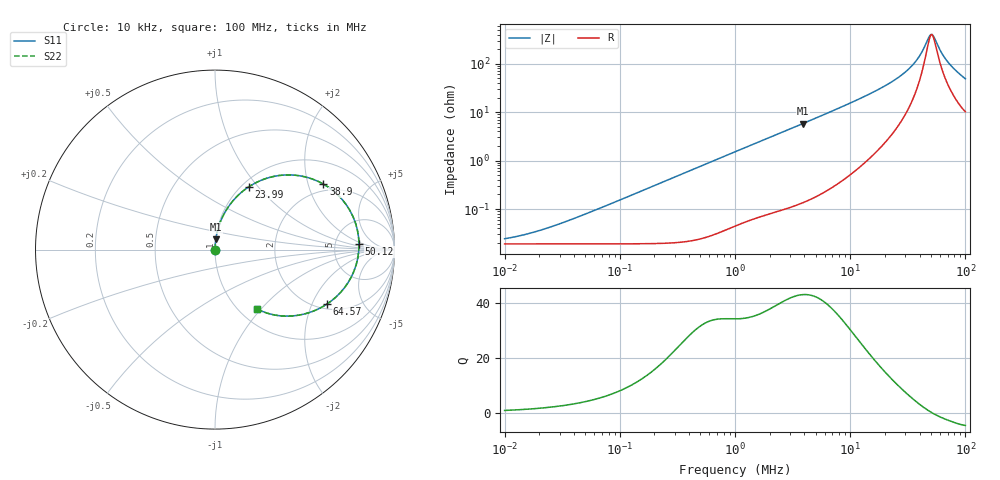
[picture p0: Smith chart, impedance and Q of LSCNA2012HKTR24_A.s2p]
! LSCNA2012HKTR24_A  S-PARAMETER MODEL  ( Standard Model )
! Model Generated by TAIYO YUDEN Corporation (http://www.ty-top.com)
! Version 2.0
! TAIYO YUDEN Control No. 171005
! Copyright(c) 2016 TAIYO YUDEN CO.,LTD. All Rights Reserved.
! Product Description (link to TY-COMPAS)
! https://ds.yuden.co.jp/TYCOMPAS/or/detail?pn=LSCNA2012HKTR24MA&u=M
! Products Name : Inductors
! Characteristics :
!  Inductance : 0.24 [uH] , SRF(min) : - [Hz] , DC Resistance(max) : 24 [mOhm]
!  Rated Current : Saturation  4.32 [A] (dL = 30 [%]), Temp Rise  3.6 [A] (dT = 40 [degC])
!  Case Size : 2.0 x 1.25 / 0.079 x 0.049 [mm/inch] , Thickness : 0.8 / 0.031 [mm/inch]
!  (Conditions: Temperature = 25 [degC] , DC Bias Current = 0 [A])
! External Node Assignments :
!  1  o---GGG---o  2
! GND o---------o GND
! Frequency Range : 10kHz  -  100MHz  [ 402 STEP ]
# MHz S RI R 50
! Freq[MHz].  S11 Real  S11 Imag  S21 Real  S21 Imag  S12 Real  S12 Imag  S22 Real  S22 Imag
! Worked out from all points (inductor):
!   401 points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, 10 kHz to 100 MHz, reference 50 ohm
!   read as one part in series: L = 242 nH near 38.02 kHz
!   highest Q = 43.1 at 3.89 MHz (marker M1), where L = 238 nH
!   self-resonance near 51.06 MHz
!   S11 on the Smith chart (normalised r, x): 10 kHz: 1.00, +0.00; 23.99 MHz: 1.08, +0.90; 38.9 MHz: 1.73, +2.52; 50.12 MHz: 8.87, +1.59; 64.57 MHz: 2.24, -2.61; 100 MHz: 1.20, -0.95
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0.01  0.00019 0.000152  0.9998 -0.000152  0.9998 -0.000152  0.00019 0.000152
0.019953  0.00019 0.000303  0.9998 -0.000303  0.9998 -0.000303  0.00019 0.000303
0.046774  0.000191 0.00071  0.9998 -0.00071  0.9998 -0.00071  0.000191 0.00071
0.218776  0.000205 0.00333  0.9998 -0.00333  0.9998 -0.00333  0.000205 0.00333
1  0.000672 0.0151  0.9993 -0.0151  0.9993 -0.0151  0.000672 0.0151
3.890451  0.00471 0.0578  0.9953 -0.0578  0.9953 -0.0578  0.00471 0.0578
4.677351  0.0065 0.0695  0.9935 -0.0695  0.9935 -0.0695  0.0065 0.0695
12.58925  0.0449 0.1879  0.9551 -0.1879  0.9551 -0.1879  0.0449 0.1879
16.98244  0.0856 0.2537  0.9144 -0.2537  0.9144 -0.2537  0.0856 0.2537
21.87762  0.1528 0.3238  0.8472 -0.3238  0.8472 -0.3238  0.1528 0.3238
23.98833  0.1904 0.3513  0.8096 -0.3513  0.8096 -0.3513  0.1904 0.3513
28.18383  0.2828 0.3956  0.7172 -0.3956  0.7172 -0.3956  0.2828 0.3956
32.35937  0.3979 0.416  0.6021 -0.416  0.6021 -0.416  0.3979 0.416
38.90451  0.6042 0.365  0.3958 -0.365  0.3958 -0.365  0.6042 0.365
44.66836  0.7514 0.2184  0.2486 -0.2184  0.2486 -0.2184  0.7514 0.2184
47.86301  0.7932 0.1102  0.2068 -0.1102  0.2068 -0.1102  0.7932 0.1102
50.11872  0.8024 0.0318  0.1976 -0.0318  0.1976 -0.0318  0.8024 0.0318
53.70318  0.7868 -0.0839  0.2132 0.0839  0.2132 0.0839  0.7868 -0.0839
58.88437  0.7205 -0.2139  0.2795 0.2139  0.2795 0.2139  0.7205 -0.2139
64.56542  0.6258 -0.3021  0.3742 0.3021  0.3742 0.3021  0.6258 -0.3021
77.62471  0.4313 -0.3695  0.5687 0.3695  0.5687 0.3695  0.4313 -0.3695
100  0.2359 -0.331  0.7641 0.331  0.7641 0.331  0.2359 -0.331
